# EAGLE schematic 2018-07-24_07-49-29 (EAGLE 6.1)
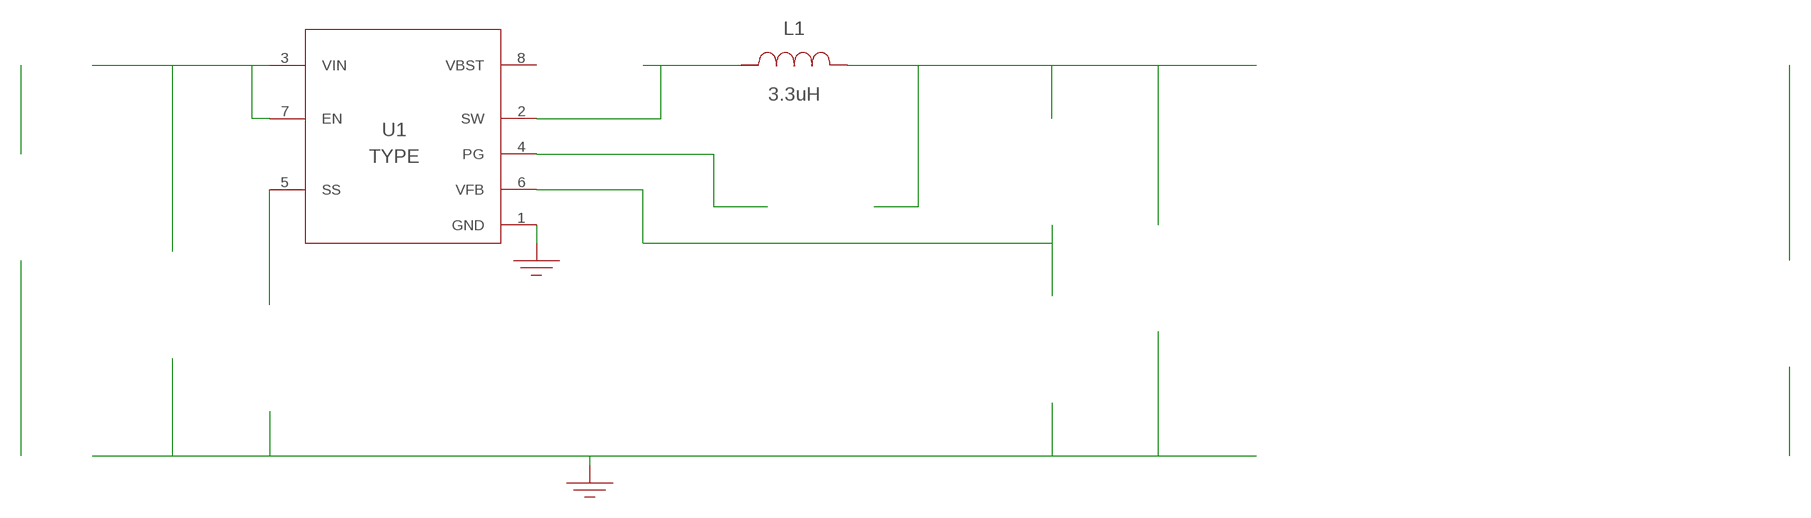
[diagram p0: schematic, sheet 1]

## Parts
CBST  100nF  C0603C104Z3VACTUC0603C104Z3VACTU  [0603]  (not placed on a sheet)
CIN  22uF  C2012X5R1V226M125ACC2012X5R1V226M125AC  [0805]  (not placed on a sheet)
COUT  22uF  C1608X5R1A226M080ACC1608X5R1A226M080AC  [0603]  (not placed on a sheet)
CSS  8.2nF  GRM033R61A822KA01DGRM033R61A822KA01D  [0201]  (not placed on a sheet)
GND  WB_GND  WB_GNDWB_GND  [WB_GND]
GND2  WB_GND  WB_GNDWB_GND  [WB_GND]
IOUT  WB_CURRENT_LOAD  WB_CURRENT_LOADWB_CURRENT_LOAD  [WB_CURRENT_LOAD]  (not placed on a sheet)
L1  3.3uH  SRR4028-3R3YSRR4028-3R3Y  [SRR4028]
RFBB  10k  RMCF0402FT10K0RMCF0402FT10K0  [0402]  (not placed on a sheet)
RFBT  33.2k  CRCW040233K2FKEDCRCW040233K2FKED  [0402]  (not placed on a sheet)
RPG  100k  ERJ-6ENF1003VERJ-6ENF1003V  [0805]  (not placed on a sheet)
U1  TPS562219DDFR  TPS562219DDFRTPS562219DDFR  [DDF0008A]
VIN  WB_BATTERY  WB_BATTERYWB_BATTERY  [WB_BATTERY]  (not placed on a sheet)

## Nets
0: Cin.2@2 Cout.2@2 Css.2@2 GND2.1 GND.1 Rfbb.2@2 U1.1(GND)
1: Cin.1@1 U1.3(VIN) U1.7(EN)
2: Rfbb.1@1 Rfbt.2@2 U1.6(VFB)
3: Rpg.2@2 U1.4(PG)
4: Cbst.1@1 L1.2 U1.2(SW)
5: Cout.1@1 L1.1 Rfbt.1@1 Rpg.1@1
6: Css.1@1 U1.5(SS)
7: Iout.+@1
8: Iout.-@2
9: Vin.+@1
10: Vin.-@2
11: Cbst.2@2 U1.8(VBST)
Unconnected: CBST.1 CBST.2 CIN.1 CIN.2 COUT.1 COUT.2 CSS.1 CSS.2 IOUT.1(+) IOUT.2(-) RFBB.1 RFBB.2 RFBT.1 RFBT.2 RPG.1 RPG.2 VIN.1(+) VIN.2(-)

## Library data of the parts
CBST = AcceleratedDesigns_Lib:C0603C104Z3VACTU; Cap: 1.0E-7; ESR: 0.0; IRMS: 0.0; Manufacturer_Name: Kemet; Manufacturer_Part_Number: C0603C104Z3VACTU; VDC: 25.0; Vendor: Kemet
CIN = AcceleratedDesigns_Lib:C2012X5R1V226M125AC; Cap: 2.2E-5; Datasheet_URL: https://product.tdk.com/en/search/capacitor/ceramic/mlcc/info?part%5Fno%3DC2012X5R1V226M125AC; ESR: 0.00205; IRMS: 4.55587; Manufacturer_Name: TDK; Manufacturer_Part_Number: C2012X5R1V226M125AC; VDC: 35.0; Vendor: TDK
COUT = AcceleratedDesigns_Lib:C1608X5R1A226M080AC; Cap: 2.2E-5; Datasheet_URL: https://product.tdk.com/en/search/capacitor/ceramic/mlcc/info?part%5Fno%3DC1608X5R1A226M080AC; ESR: 0.00371; IRMS: 2.69936; Manufacturer_Name: TDK; Manufacturer_Part_Number: C1608X5R1A226M080AC; VDC: 10.0; Vendor: TDK
CSS = AcceleratedDesigns_Lib:GRM033R61A822KA01D; Cap: 8.2E-9; ESR: 0.0; IRMS: 0.0; Manufacturer_Name: MuRata; Manufacturer_Part_Number: GRM033R61A822KA01D; VDC: 10.0; Vendor: MuRata
GND GND2 = AcceleratedDesigns_Lib:WB_GND; Manufacturer_Name: WB_GND; Manufacturer_Part_Number: WB_GND; PowerPortType: POWER_GROUND; Value: Value
IOUT = AcceleratedDesigns_Lib:WB_CURRENT_LOAD; Manufacturer_Name: WB_CURRENT_LOAD; Manufacturer_Part_Number: WB_CURRENT_LOAD; PowerPortType: POWER_GROUND; Value: Value
L1 = AcceleratedDesigns_Lib:SRR4028-3R3Y; DCR: 0.035; IDC: 2.15; L: 3.3E-6; Manufacturer_Name: Bourns; Manufacturer_Part_Number: SRR4028-3R3Y; Vendor: Bourns
RFBB = AcceleratedDesigns_Lib:RMCF0402FT10K0; Datasheet_URL: https://www.seielect.com/Catalog/SEI%2DRMCF%5FRMCP.pdf; Manufacturer_Name: Stackpole Electronics Inc; Manufacturer_Part_Number: RMCF0402FT10K0; Power: 0.063; Resistance: 10000.0; Tolerance: 1.0; Vendor: Stackpole Electronics Inc
RFBT = AcceleratedDesigns_Lib:CRCW040233K2FKED; Manufacturer_Name: Vishay-Dale; Manufacturer_Part_Number: CRCW040233K2FKED; Power: 0.063; Resistance: 33200.0; Tolerance: 1.0; Vendor: Vishay-Dale
RPG = AcceleratedDesigns_Lib:ERJ-6ENF1003V; Manufacturer_Name: Panasonic; Manufacturer_Part_Number: ERJ-6ENF1003V; Power: 0.125; Resistance: 100000.0; Tolerance: 1.0; Vendor: Panasonic
U1 = AcceleratedDesigns_Lib:TPS562219DDFR; CompType: IC; Manufacturer: Texas Instruments; Manufacturer_Name: Texas Instruments; Manufacturer_Part_Number: TPS562219DDFR; MountType: SMT; PIN_COUNT: 8; PackageReference: DDF0008A; PartNumber: TPS562219DDF; RefDes: RefDes; RoHS: Y; TYPE: TYPE; Value: Value
VIN = AcceleratedDesigns_Lib:WB_BATTERY; Manufacturer_Name: WB_BATTERY; Manufacturer_Part_Number: WB_BATTERY; PowerPortType: POWER_GROUND; Value: Value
